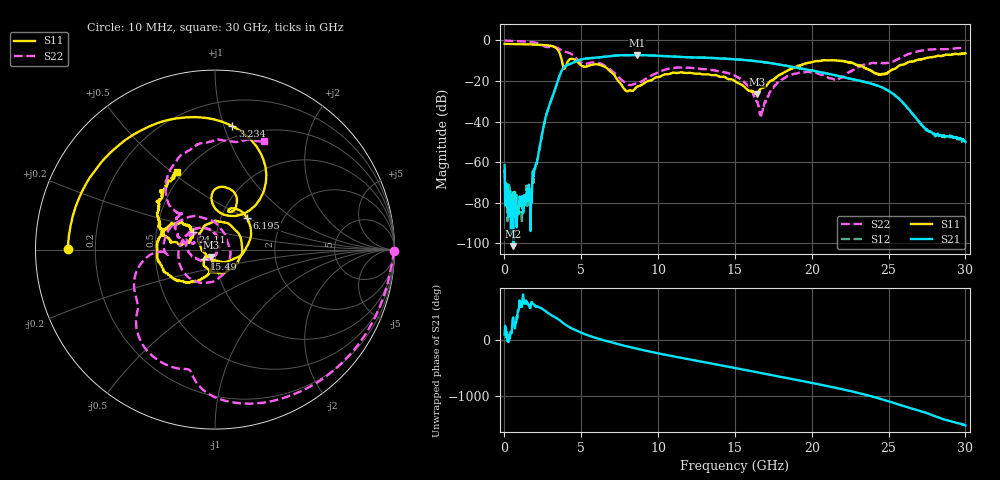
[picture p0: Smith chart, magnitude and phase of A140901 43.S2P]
!  2-Port S-parameters saved by WinCal
! VAR MeasName=S-Parameters (CALIBRATED_DATA) read from VNA (N5244A)
! VAR MeasDate=11/3/2014 9:33:59 AM
! VAR NAME=A140901 43
! VAR FILENAME=A140901 43.S2P
! VAR DATE=11/3/2014 9:33:59 AM
! VAR PHYS_PORTS=1,2
# Hz S RI R 50
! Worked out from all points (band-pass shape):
!   801 points, 10 MHz to 30 GHz, reference 50 ohm
!   highest |S21| = -7.18 dB at 8.632 GHz (marker M1); lowest = -101.4 dB at 572.3 MHz (marker M2)
!   |S21| within 3 dB of the highest: 4.703 GHz to 16.28 GHz (11.58 GHz wide, 110 % of centre)
!   lowest |S11| = -26.5 dB at 16.43 GHz (marker M3), VSWR 1.10, Z = 47.7 - j4.07 ohm
!   |S11| at or under -10 dB: 3.735 GHz to 4.16 GHz (425.1 MHz wide, 10.8 % of centre); 4.679 GHz to 20.63 GHz (15.95 GHz wide, 126 % of centre); 21.79 GHz to 26.73 GHz (4.934 GHz wide, 20.3 % of centre)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
!   |S22| runs from -38.3 to 0.0 dB; largest |S21 - S12| = 0.0035
!   S11 on the Smith chart (normalised r, x): 10 MHz: 0.10, +0.00; 3.234 GHz: 0.40, +1.07; 6.195 GHz: 1.32, +0.50; 15.49 GHz: 0.88, -0.09; 24.11 GHz: 0.77, +0.16; 30 GHz: 0.47, +0.52
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1e7  -0.8191 0.00313  -0.000178 0.000818  -0.000256 0.000609  0.998 -0.00825
5.723125e8  -0.7927 0.1855  5.73e-06 6.26e-06  6.33e-05 0.00019  0.9041 -0.3513
1.621962e9  -0.6255 0.4952  -9.47e-05 -0.000182  -0.000182 -0.000101  0.4544 -0.7996
3.233925e9  0.0962 0.6877  0.0285 0.0456  0.0285 0.0454  -0.3283 -0.6079
4.096138e9  -0.0201 0.288  -0.0755 -0.2367  -0.075 -0.2367  -0.4445 -0.2487
5.033325e9  0.1008 0.2141  -0.2141 0.2671  -0.2142 0.2668  -0.2728 -0.0178
6.195438e9  0.1781 0.1775  0.3649 0.1186  0.3638 0.119  -0.2444 0.1269
7.470012e9  0.0651 -0.0669  0.088 -0.4201  0.0889 -0.4208  0.0319 0.1158
8.632125e9  -0.072 -0.00682  -0.3978 -0.1818  -0.3976 -0.1817  0.0866 -0.0184
1.001916e10  -0.0844 0.0934  -0.2228 0.3546  -0.2215 0.3539  0.0116 -0.1652
1.23059e10  0.1471 0.0471  0.3815 0.00468  0.3808 0.00558  -0.2042 -0.042
1.5005e10  -0.063 -0.0754  -0.2608 -0.2206  -0.2613 -0.2207  -0.0565 0.1206
1.549234e10  -0.0601 -0.0515  -0.3213 -0.0825  -0.3224 -0.0827  -0.0141 0.1003
1.642952e10  -0.0213 -0.0425  -0.2481 0.1768  -0.2486 0.1768  0.0265 0.016
1.672942e10  -0.0152 -0.0647  -0.1838 0.2326  -0.1839 0.2327  0.0109 -0.0118
1.789154e10  -0.0371 -0.1363  0.1021 0.232  0.102 0.2336  -0.0778 -0.06
2.002832e10  -0.2581 -0.14  0.1219 -0.134  0.1227 -0.1342  -0.1395 0.0751
2.164029e10  -0.3124 0.0565  -0.103 -0.0878  -0.1032 -0.0872  -0.0923 0.0526
2.411446e10  -0.1236 0.0992  0.0449 0.0669  0.0449 0.0675  -0.2077 0.1839
2.501416e10  -0.1594 0.0369  0.0538 -0.0172  0.0541 -0.0169  -0.1963 0.2053
2.756331e10  -0.3214 0.1946  -0.00351 0.0047  -0.00338 0.00495  -0.1021 0.5821
3e10  -0.2089 0.4301  8.11e-05 -0.00313  -9.24e-05 -0.00294  0.2706 0.6037
